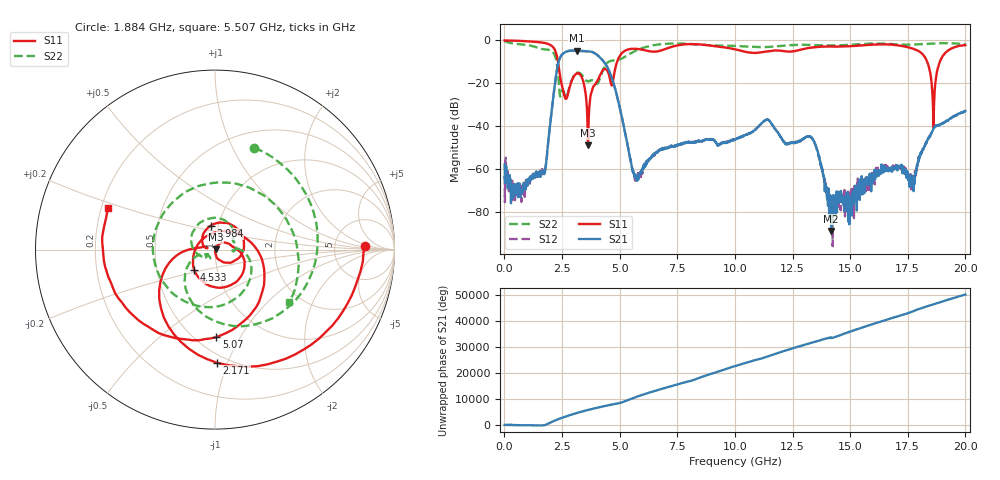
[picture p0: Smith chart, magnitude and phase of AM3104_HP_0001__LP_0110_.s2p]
!Created with skrf (http://scikit-rf.org).
# Hz S RI R 50.0
!freq ReS11 ImS11 ReS21 ImS21 ReS12 ImS12 ReS22 ImS22
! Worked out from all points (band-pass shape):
!   1601 points, 10 MHz to 20 GHz, reference 50 ohm
!   highest |S21| = -4.71 dB at 3.133 GHz (marker M1); lowest = -89.0 dB at 14.18 GHz (marker M2)
!   |S21| within 3 dB of the highest: 2.43 GHz to 4.125 GHz (1.695 GHz wide, 51.7 % of centre)
!   lowest |S11| = -49.1 dB at 3.633 GHz (marker M3), VSWR 1.01, Z = 50.3 + j0.21 ohm
!   |S11| at or under -10 dB: 2.325 GHz to 4.889 GHz (2.564 GHz wide, 71.1 % of centre); 18.34 GHz to 18.89 GHz (542.4 MHz wide, 2.91 % of centre)
!   |S22| runs from -26.5 to -0.2 dB; largest |S21 - S12| = 0.0038
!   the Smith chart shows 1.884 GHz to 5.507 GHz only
!   S11 on the Smith chart (normalised r, x): 1.884 GHz: 11, +1; 2.171 GHz: 0.44, -0.92; 2.984 GHz: 0.92, +0.25; 4.533 GHz: 0.77, -0.18; 5.07 GHz: 0.62, -0.80; 5.507 GHz: 0.23, +0.18
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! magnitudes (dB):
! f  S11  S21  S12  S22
! 10 MHz  0.0  -58.0  -63.2  -0.2
! 709.6 MHz  -0.2  -73.0  -71.8  -1.8
! 1.884 GHz  -1.6  -49.3  -49.2  -4.3
! 2.171 GHz  -4.0  -22.2  -22.1  -6.6
! 2.634 GHz  -26.7  -5.5  -5.5  -25.6
! 2.984 GHz  -17.4  -4.7  -4.7  -17.0
! 3.133 GHz  -15.5  -4.7  -4.7  -15.3
! 3.346 GHz  -16.9  -4.9  -4.9  -15.9
! 3.633 GHz  -49.1  -5.1  -5.1  -19.0
! 4.533 GHz  -15.8  -13.9  -13.9  -9.9
! 5.07 GHz  -6.2  -34.4  -34.4  -8.5
! 5.507 GHz  -3.9  -57.7  -57.8  -5.9
! 6.682 GHz  -5.0  -51.4  -51.7  -1.9
! 10.01 GHz  -4.1  -46.1  -46.4  -2.5
! 11.39 GHz  -5.1  -36.9  -36.9  -3.0
! 13.34 GHz  -3.3  -45.6  -45.7  -2.2
! 14.18 GHz  -2.8  -89.0  -78.4  -2.3
! 16.68 GHz  -1.9  -60.0  -59.8  -1.6
! 17.71 GHz  -3.8  -63.9  -66.1  -1.9
! 18.61 GHz  -40.7  -41.2  -41.2  -1.4
! 19.03 GHz  -7.1  -38.6  -38.6  -1.3
! 20 GHz  -2.2  -33.0  -33.0  -1.7
